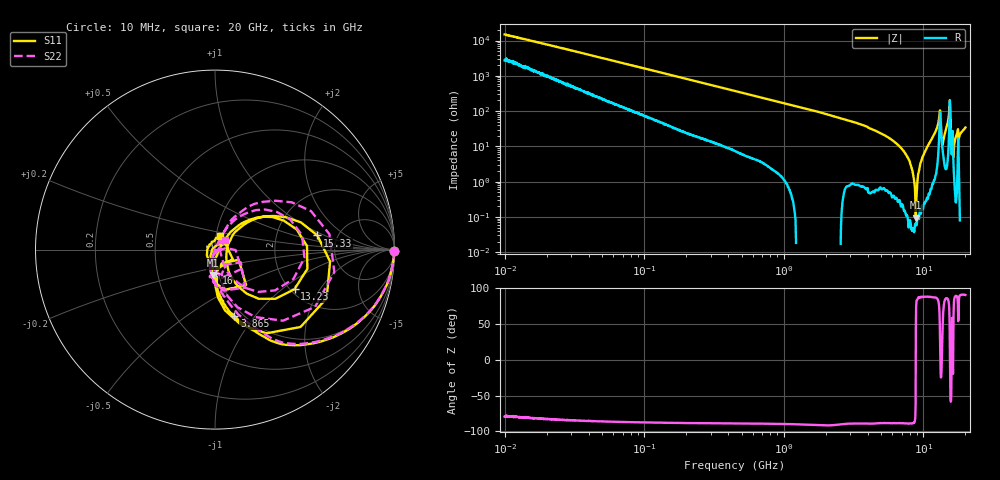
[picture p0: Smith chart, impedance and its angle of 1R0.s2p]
!Keysight Technologies,P5008B,MY61100088,A.16.20.02
!Date: Monday, October 30, 2023 16:06:44
!Correction: S11(C  2-Port  )
!S21(C  2-Port  )
!S12(C  2-Port  )
!S22(C  2-Port  )
!S2P File: Measurements: S11, S21, S12, S22:Log Frequency Sweep
# Hz S  dB  R 50
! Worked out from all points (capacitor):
!   1601 points, 10 MHz to 20 GHz, reference 50 ohm
!   read as one part in series: C = 1.07 pF near 10.39 MHz
!   lowest |Z| = 95.4 mohm at 8.834 GHz (marker M1)
!   series resonance near 8.82 GHz, so ESL is about 300 pH
!   S11 on the Smith chart (normalised r, x): 10 MHz: open; 3.865 GHz: 0.91, -0.79; 13.23 GHz: 2.11, -1.23; 15.33 GHz: 3.50, +0.83; 16 GHz: 0.98, -0.26; 20 GHz: 1.05, +0.15
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1e7  -0.01 -0.4  -43.43 79.1  -43.41 79.2  -0.01 -0.4
3.555162e7  -0.02 -1.3  -32.96 83.8  -32.96 83.8  -0.02 -1.3
1.263918e8  -0.06 -4.6  -22.25 83.2  -22.26 83.2  -0.06 -4.5
4.472136e8  -0.36 -15.7  -11.75 73.3  -11.75 73.3  -0.36 -15.4
1.589917e9  -2.63 -45.5  -3.32 45.7  -3.32 45.7  -2.64 -44.8
3.865292e9  -8.27 -73.8  -0.77 17.4  -0.77 17.3  -8.26 -70.1
5.652411e9  -12.21 -85.0  -0.29 5.3  -0.30 5.3  -12.23 -81.5
8.834242e9  -16.90 -95.2  -0.08 -8.2  -0.08 -8.3  -17.03 -99.1
1.048196e10  -21.83 -93.9  -0.02 -14.4  -0.03 -14.5  -21.73 -106.0
1.147208e10  -33.08 -34.6  -0.03 -19.1  -0.03 -19.1  -41.30 -111.4
1.180378e10  -27.75 31.2  -0.05 -21.1  -0.06 -21.2  -30.08 66.4
1.273595e10  -11.86 40.7  -0.66 -32.8  -0.66 -32.8  -12.05 51.2
1.322929e10  -6.11 -26.4  -5.55 -13.0  -5.55 -13.0  -6.62 -20.5
1.380717e10  -19.97 -48.6  -0.52 -15.4  -0.52 -15.4  -23.49 -52.5
1.413906e10  -23.18 10.4  -0.23 -20.9  -0.23 -21.0  -26.14 49.2
1.482695e10  -12.58 39.9  -0.46 -33.0  -0.46 -33.0  -12.59 57.1
1.53283e10  -4.79 7.9  -4.07 -52.1  -4.07 -52.2  -4.78 21.8
1.599787e10  -17.58 -87.8  -0.60 -14.7  -0.60 -14.7  -17.01 -74.3
1.709804e10  -27.77 -127.3  -0.08 -24.1  -0.09 -24.2  -28.00 -109.7
1.818725e10  -25.32 -147.3  -0.09 -27.6  -0.10 -27.6  -24.49 -100.7
1.898171e10  -28.37 152.9  -0.04 -32.6  -0.04 -32.6  -35.23 -65.1
2e10  -22.07 69.0  -0.03 -37.7  -0.03 -37.7  -22.55 43.8
